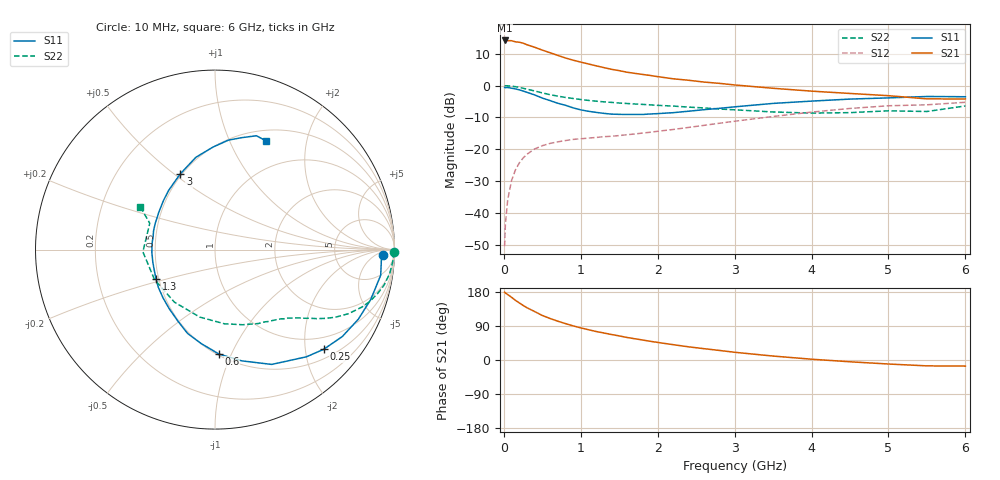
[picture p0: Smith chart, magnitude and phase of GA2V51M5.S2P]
! Infineon Technologies  Discrete & RF Semiconductors
! BF775
! Si NPN RF Bipolar Junction Transistor in SOT23
! VCE = 2.5 V  IC = 1.5 mA
! Common Emitter S-Parameters:  May  1996
# GHz  S  MA  R  50
!  f  S11  S21  S12  S22
! GHz  MAG  ANG  MAG  ANG  MAG  ANG  MAG  ANG
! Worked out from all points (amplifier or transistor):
!   36 points, 10 MHz to 6 GHz, reference 50 ohm
!   highest |S21| = 14.2 dB at 10 MHz (marker M1)
!   |S21| within 3 dB of that: start of sweep to 496.5 MHz
!   unconditionally stable (mu >= 1): 1.266 GHz to 4.235 GHz; 5.058 GHz to end of sweep
!   at 250 MHz: K = 0.25, MSG = 18.1 dB, |S12| = -22.8 dB
!   at 1.4 GHz: K = 1.08, MAG = 8.8 dB, |S12| = -15.9 dB
!   at 6 GHz: K = 1.03, MAG = -0.5 dB, |S12| = -5.2 dB
!   S11 on the Smith chart (normalised r, x): 10 MHz: 25, -11; 250 MHz: 0.70, -2.40; 600 MHz: 0.51, -0.90; 1.3 GHz: 0.48, -0.18; 3 GHz: 0.49, +0.53; 6 GHz: 0.63, +1.38
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0.01  0.9338 -1.7  5.125 178.9  0.003 88.6  0.999 -0.8
0.02  0.9286 -3.4  5.031 176.9  0.0066 86.6  0.9953 -1.6
0.05  0.9343 -8.8  5.085 172.7  0.016 84.9  0.9924 -4.0
0.1  0.9111 -17.8  5.079 165.5  0.0322 79.3  0.9819 -8.0
0.15  0.8878 -25.9  4.883 157.6  0.0471 74.1  0.9625 -11.9
0.2  0.8591 -34.3  4.811 150.8  0.0607 69.6  0.9378 -15.2
0.25  0.8219 -42.5  4.65 144.1  0.0727 65.0  0.9097 -18.5
0.3  0.7853 -49.5  4.39 138.0  0.0834 61.6  0.88 -21.3
0.4  0.7136 -63.7  4.009 127.9  0.1011 55.1  0.8242 -25.7
0.5  0.6379 -76.4  3.615 117.5  0.1138 49.9  0.7684 -29.4
0.6  0.582 -87.9  3.288 109.6  0.1235 46.0  0.7213 -32.1
0.8  0.4917 -108.1  2.721 96.1  0.137 41.0  0.6523 -35.9
0.9  0.4479 -117.7  2.511 90.1  0.1428 39.6  0.6284 -37.5
1.1  0.3951 -137.1  2.19 79.9  0.1498 38.4  0.5856 -40.5
1.3  0.3666 -153.9  1.919 71.3  0.1575 38.2  0.556 -43.4
1.7  0.3526 175.2  1.56 56.1  0.1737 39.6  0.5145 -49.7
2.2  0.3756 146.6  1.281 40.5  0.2045 42.1  0.4773 -59.7
3  0.4642 114.6  1.025 20.4  0.2755 41.6  0.4169 -82.7
3.5  0.5253 101.7  0.908 10.4  0.3275 38.0  0.3854 -102.7
4.5  0.6145 83.0  0.753 -4.7  0.4379 26.3  0.3762 -153.8
5.5  0.675 70.0  0.619 -15.5  0.4996 10.2  0.392 158.0
6  0.6688 64.6  0.617 -16.1  0.5472 5.8  0.4795 150.2
